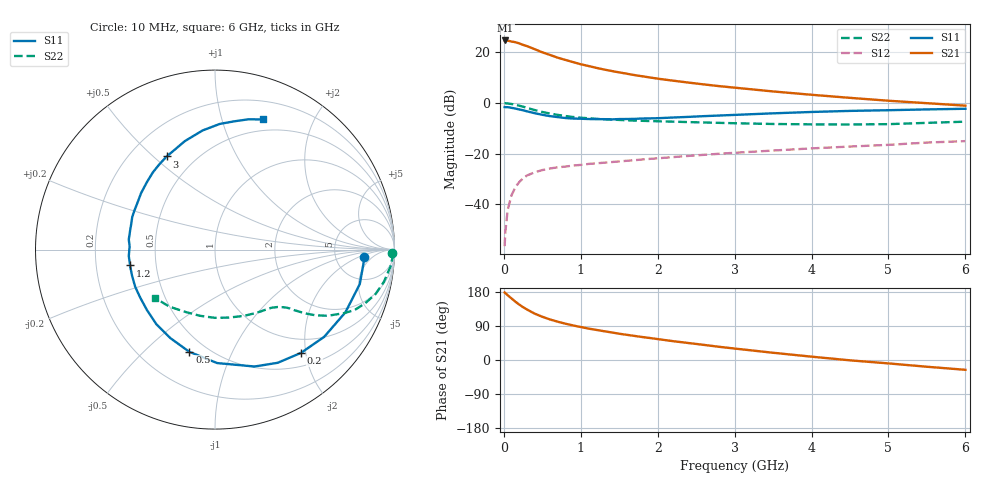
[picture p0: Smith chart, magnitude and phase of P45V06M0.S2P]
! SIEMENS Small Signal Semiconductors
! BFP182
! Si NPN RF Bipolar Junction Transistor in SOT143
! VCE = 5 V  IC = 6 mA
! Common Emitter S-Parameters:  March  1996
# GHz  S  MA  R  50
!  f  S11  S21  S12  S22
! GHz  MAG  ANG  MAG  ANG  MAG  ANG  MAG  ANG
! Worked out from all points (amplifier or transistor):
!   36 points, 10 MHz to 6 GHz, reference 50 ohm
!   highest |S21| = 24.7 dB at 20 MHz (marker M1)
!   |S21| within 3 dB of that: start of sweep to 364.6 MHz
!   unconditionally stable (mu >= 1): 1.521 GHz to 5.593 GHz
!   at 250 MHz: K = 0.22, MSG = 26.3 dB, |S12| = -29.7 dB
!   at 1.4 GHz: K = 0.96, MSG = 18.0 dB, |S12| = -23.3 dB
!   at 6 GHz: K = 0.96, MSG = 7.0 dB, |S12| = -15.0 dB
!   lowest NFmin = 1.25 dB at 450 MHz
!   S11 on the Smith chart (normalised r, x): 10 MHz: 10, -3; 200 MHz: 0.73, -1.91; 500 MHz: 0.40, -0.70; 1.2 GHz: 0.35, -0.08; 3 GHz: 0.35, +0.55; 6 GHz: 0.38, +1.36
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0.01  0.8335 -2.7  16.97 178.2  0.0015 82.3  0.9883 -1.1
0.02  0.831 -5.3  17.21 176.7  0.0029 82.5  0.9911 -2.2
0.05  0.8292 -13.4  17.09 170.9  0.0078 85.7  0.9826 -5.4
0.1  0.8062 -25.7  16.39 162.4  0.0152 74.7  0.9587 -10.7
0.15  0.7787 -38.6  15.91 153.9  0.0218 69.7  0.9281 -15.5
0.2  0.7489 -50.2  15.07 146.3  0.0276 64.8  0.8883 -19.7
0.25  0.721 -61.0  14.08 139.4  0.0327 61.1  0.8487 -23.3
0.3  0.6877 -71.3  13.32 133.4  0.0372 56.6  0.8054 -26.0
0.4  0.6323 -88.9  11.61 122.4  0.043 49.8  0.7286 -30.4
0.5  0.5872 -104.1  10.04 114.1  0.0476 45.1  0.6683 -33.2
0.6  0.5522 -116.8  8.911 107.0  0.0512 42.6  0.6222 -35.0
0.7  0.5286 -128.2  7.869 101.1  0.054 40.5  0.5851 -36.3
0.8  0.5071 -138.4  7.11 95.8  0.0558 39.2  0.5551 -37.4
1.1  0.4844 -162.7  5.392 82.9  0.0629 37.0  0.5011 -39.9
1.2  0.4814 -169.4  4.96 79.5  0.0648 36.3  0.4899 -40.9
1.7  0.4881 163.0  3.567 63.5  0.0747 36.5  0.4505 -46.1
2.2  0.5186 142.5  2.768 49.7  0.0859 35.8  0.4295 -53.1
3  0.5846 117.4  2.016 30.2  0.1045 33.2  0.4004 -67.6
3.5  0.6274 105.5  1.696 19.1  0.1157 30.6  0.3868 -78.3
4.5  0.7008 87.8  1.268 -0.9  0.1387 25.0  0.3782 -102.9
5.5  0.7501 75.5  0.995 -17.8  0.1663 19.4  0.407 -128.7
6  0.772 69.9  0.889 -25.9  0.1776 15.0  0.4295 -141.2
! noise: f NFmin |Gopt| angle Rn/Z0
0.45  1.25  0.25  39  0.3
0.9  1.4  0.25  78  0.23
1.8  1.95  0.21  151  0.2
